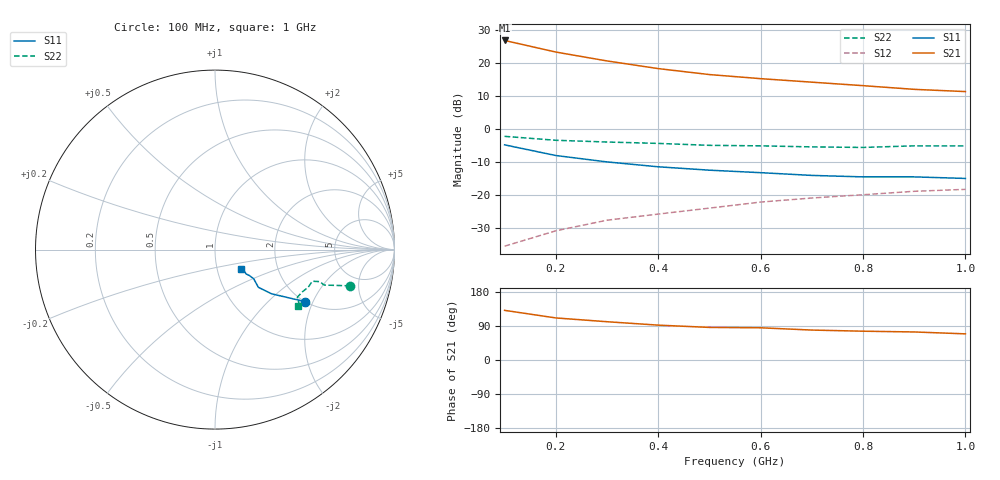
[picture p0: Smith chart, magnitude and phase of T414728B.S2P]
!AT-41472
!S-PARAMETERS at Vce=8V  Ic=25mA.  LAST UPDATED 07-21-92
# ghz s ma r 50
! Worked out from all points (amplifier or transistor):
!   10 points, 100 MHz to 1 GHz, reference 50 ohm
!   highest |S21| = 26.9 dB at 100 MHz (marker M1)
!   |S21| within 3 dB of that: start of sweep to 185.5 MHz
!   unconditionally stable (mu >= 1): 384.8 MHz to end of sweep
!   at 200 MHz: K = 0.85, MSG = 27.0 dB, |S12| = -30.8 dB
!   at 600 MHz: K = 1.04, MAG = 17.5 dB, |S12| = -22.0 dB
!   at 1 GHz: K = 1.04, MAG = 13.5 dB, |S12| = -18.2 dB
0.1  0.58 -30.0  22.02 131.0  0.017 78.0  0.78 -15.0
0.2  0.4 -38.0  14.7 111.0  0.029 80.0  0.68 -17.0
0.3  0.32 -41.0  10.79 101.0  0.042 79.0  0.64 -18.0
0.4  0.27 -37.0  8.26 92.0  0.052 76.0  0.61 -17.0
0.5  0.24 -37.0  6.71 86.0  0.064 73.0  0.57 -18.0
0.6  0.22 -38.0  5.82 85.0  0.079 74.0  0.56 -22.0
0.7  0.2 -36.0  5.15 79.0  0.091 72.0  0.54 -26.0
0.8  0.19 -35.0  4.56 76.0  0.102 71.0  0.53 -30.0
0.9  0.19 -38.0  4.01 74.0  0.115 72.0  0.56 -33.0
1  0.18 -37.0  3.71 69.0  0.123 69.0  0.56 -34.0
